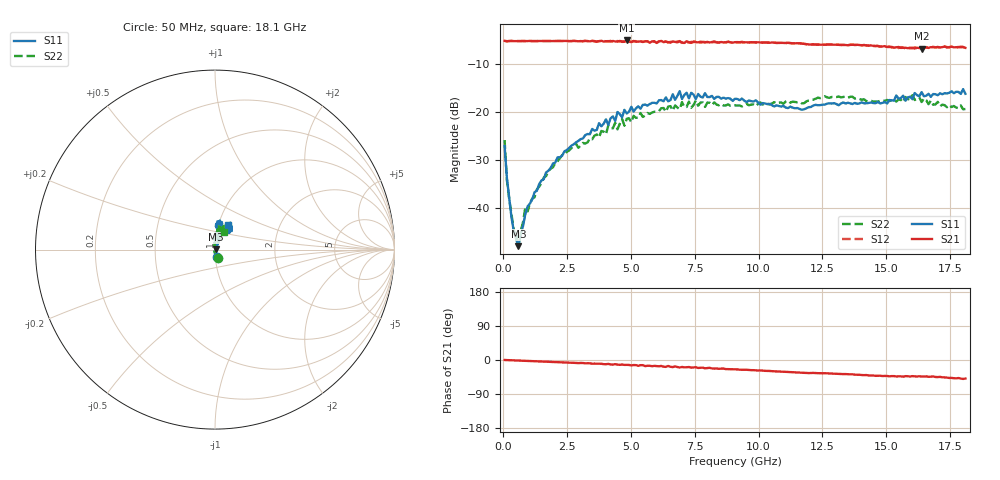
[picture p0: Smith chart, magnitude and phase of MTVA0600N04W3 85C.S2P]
! Network Analyzer HP8720D.06.14 Serial No. US36140669
!  8 Jul 2005  11:48:57
! Frequency  S11  S21  S12  S22
# HZ  S  DB R 50
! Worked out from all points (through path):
!   201 points, 50 MHz to 18.1 GHz, reference 50 ohm
!   highest |S21| = -5.15 dB at 4.833 GHz (marker M1); lowest = -6.8 dB at 16.39 GHz (marker M2)
!   group delay of S21, straight-line fit = 7.67 ps
!   lowest |S11| = -47.9 dB at 591.5 MHz (marker M3), VSWR 1.01, Z = 50.4 + j0.111 ohm
!   |S11| at or under -10 dB: start of sweep to end of sweep
!   |S22| runs from -46.5 to -16.5 dB; largest |S21 - S12| = 0.022
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5e7  -27.07 -76.5  -5.22 0.0  -5.25 0.3  -25.85 -71.7
1.4025e8  -33.77 -70.1  -5.32 -0.2  -5.30 -0.3  -34.19 -94.2
2.305e8  -37.80 -62.7  -5.27 -0.5  -5.26 -0.6  -38.14 -108.2
5.0125e8  -46.40 -12.8  -5.28 -1.4  -5.27 -1.3  -46.55 -167.9
5.915e8  -47.89 15.8  -5.25 -1.3  -5.28 -1.4  -45.02 168.1
6.8175e8  -45.47 35.5  -5.28 -1.7  -5.27 -1.8  -44.75 150.9
8.6225e8  -41.21 49.0  -5.27 -2.1  -5.28 -2.1  -39.79 140.9
9.525e8  -39.60 55.7  -5.27 -2.3  -5.26 -2.4  -40.68 123.6
1.6745e9  -32.57 62.0  -5.26 -4.3  -5.26 -4.4  -33.34 99.3
3.1185e9  -25.51 70.3  -5.29 -8.0  -5.31 -8.3  -26.44 95.1
4.47225e9  -20.01 68.4  -5.37 -12.2  -5.26 -11.4  -23.63 92.5
4.83325e9  -20.31 78.2  -5.15 -12.8  -5.30 -13.6  -21.43 81.0
6.09675e9  -17.58 75.3  -5.35 -16.7  -5.28 -16.6  -19.82 81.4
6.909e9  -15.67 80.7  -5.27 -19.8  -5.41 -18.5  -19.43 75.1
6.99925e9  -17.32 80.1  -5.57 -18.4  -5.65 -20.0  -17.96 76.9
7.36025e9  -16.02 75.7  -5.66 -20.2  -5.45 -19.3  -19.13 81.7
7.54075e9  -17.33 78.1  -5.48 -19.0  -5.35 -21.2  -17.60 80.6
9.075e9  -17.26 85.7  -5.51 -24.6  -5.48 -24.7  -18.64 71.3
1.21435e10  -18.67 74.6  -5.97 -34.1  -5.93 -34.3  -17.45 68.8
1.512175e10  -17.52 51.6  -6.51 -43.1  -6.37 -42.7  -17.73 69.4
1.638525e10  -15.90 55.0  -6.82 -43.5  -6.63 -42.9  -17.94 64.1
1.81e10  -16.22 62.7  -6.68 -49.0  -6.80 -49.9  -19.39 63.3
